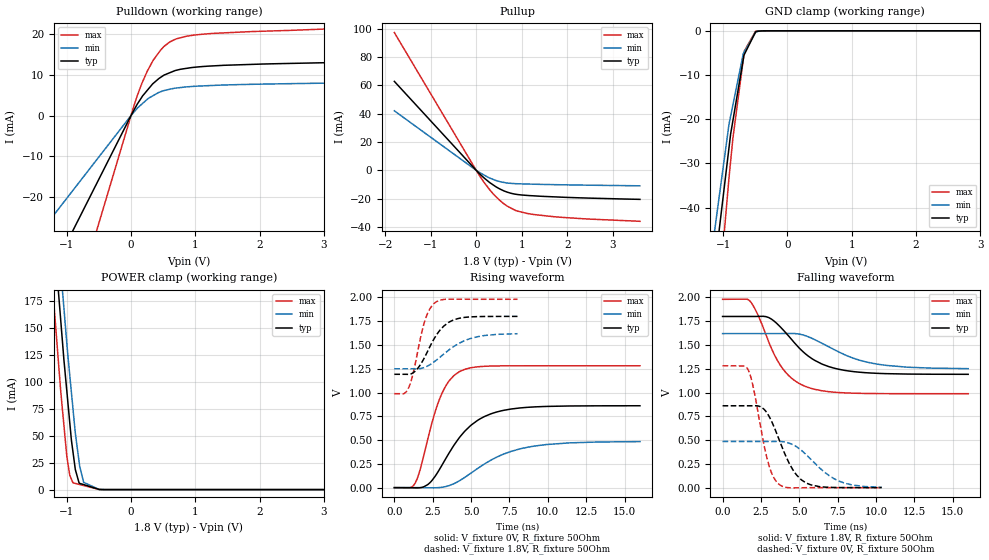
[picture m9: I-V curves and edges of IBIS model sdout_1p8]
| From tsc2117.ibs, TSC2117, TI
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|   sdout_1p8 Model
[Model]   sdout_1p8
Model_type   3-state
Polarity   Non-Inverting
Vmeas = 0.9
Vref = 0.9
Cref = 10pF
Rref = 50
|   typ   min   max
|   (nom PVT)   (fast PVT)   (slow PVT)
|C_comp from frequency sweep method (F=25MHz)
|C_comp   4.331e-12   4.023e-12   4.384e-12
|ON state : BUFFER OUTPUT TURNED HIGH
|C_comp   4.331e-12   4.023e-12   4.384e-12
|OFF state: BUFFER IN HIGH IMPEDANCE
|C_comp   1.705e-12   1.701e-12   1.707e-12
|C_comp from LC tank measurement(L=1nH)
|Resonant Frequency(Hz)   4.060e+09   4.120e+09   4.000e+09
C_comp   1.538e-12   1.494e-12   1.585e-12
|ON state : BUFFER OUTPUT TURNED HIGH
|Resonant Frequency(Hz)   4.060e+09   4.120e+09   4.000e+09
|C_comp   1.538e-12   1.494e-12   1.585e-12
|OFF state: BUFFER IN HIGH IMPEDANCE
|Resonant Frequency(Hz)   4.240e+09   4.260e+09   4.238e+09
|C_comp   1.410e-12   1.397e-12   1.411e-12
| Where nom  PVT is Nominal Process, 1.8V, 48C
|   Fast PVT is Strong Process,  1.98V, -40C
|   Slow PVT is Weak Process,   1.62V, 108C
[Voltage Range]   1.8   1.62   1.98
|Ambient Temperature   25   85   -40
|Junction Temperature
[Temperature Range]   48   108   -40
[Pullup Reference]   1.8   1.62   1.98
[Pulldown Reference]   0   0   0
[Power Clamp Reference]   1.8   1.62   1.98
[GND Clamp Reference]   0   0   0
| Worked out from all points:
|   slope of the pulldown table from 0 to 0.27 V, typ, clamps not added: 41.3 ohm
|   slope of the pullup table from 0 to 0.27 V, typ, clamps not added: 34 ohm
|   GND clamp passes 1 mA (typ) near -0.52 V on its own axis
|   POWER clamp passes 1 mA (typ) near -0.54 V on its own axis
|   falling waveform, V_fixture 1.8V, R_fixture 50Ohm: 20-80 % time 2.48ns typ, 3.15ns min, 1.86ns max; typ from 1.8 V to 1.19 V
|   rising waveform, V_fixture 0V, R_fixture 50Ohm: 20-80 % time 2.4ns typ, 3.26ns min, 1.41ns max; typ from 0 V to 0.861 V
|   rising waveform, V_fixture 1.8V, R_fixture 50Ohm: 20-80 % time 1.33ns typ, 1.97ns min, 843ps max; typ from 1.19 V to 1.8 V
|   falling waveform, V_fixture 0V, R_fixture 50Ohm: 20-80 % time 1.43ns typ, 2.05ns min, 947ps max; typ from 0.861 V to 0 V
[Pulldown]
|   Voltage   I(typ)   I(min)   I(max)
-1.8V     -56.49mA   -36.75mA   -95.55mA
-72mV     -2.259mA   -1.47mA    -3.822mA
95.04mV   2.758mA    1.751mA    4.798mA
168.3mV   4.552mA    2.822mA    7.911mA
251.5mV   6.192mA    3.988mA    10.89mA
348.5mV   7.968mA    4.952mA    13.71mA
463.3mV   9.448mA    5.897mA    16.21mA
601.9mV   10.55mA    6.481mA    18.13mA
698.9mV   11.15mA    6.779mA    18.88mA
855.4mV   11.62mA    7.059mA    19.53mA
1.277V    12.25mA    7.427mA    20.26mA
3.6V      13.28mA    8.129mA    21.69mA
[GND Clamp]
|   Voltage   I(typ)   I(min)   I(max)
-1.8V     -205.1mA   -122.8mA   -348.8mA
-1.168V   -58.11mA   -49.06mA   -76.74mA
-910.4mV  -26.61mA   -21.27mA   -33.47mA
-883.8mV  -23.38mA   -19.33mA   -29.52mA
-847.4mV  -20.24mA   -16.71mA   -24.19mA
-686.9mV  -6.4mA     -5.151mA   -6.472mA
-676.8mV  -5.531mA   -4.896mA   -5.359mA
-669.2mV  -5.311mA   -4.704mA   -4.525mA
-495mV    -237uA     -292.7uA   -66.28uA
-309.4mV  -2.036uA   -3.46uA    -90.99nA
3.6V      0A         0A         0A
[Pullup]
|   Voltage   I(typ)   I(min)   I(max)
-1.8V     62.74mA    41.98mA    97.18mA
95.04mV   -3.093mA   -1.942mA   -4.857mA
348.5mV   -9.775mA   -6.119mA   -15.69mA
601.9mV   -14.42mA   -8.513mA   -23.45mA
683.1mV   -15.42mA   -8.991mA   -25.3mA
900.9mV   -17.04mA   -9.476mA   -28.73mA
1.277V    -18.04mA   -9.812mA   -31.23mA
2.376V    -19.52mA   -10.46mA   -34.22mA
3.6V      -20.5mA    -10.94mA   -35.98mA
[POWER Clamp]
|   Voltage   I(typ)   I(min)   I(max)
-1.8V     718.4mA    754.7mA    668.7mA
-1.215V   248.1mA    295.1mA    184.9mA
-1.131V   185.5mA    231.6mA    120.5mA
-1.044V   121.1mA    169.1mA    60.29mA
-999.9mV  92.81mA    137.3mA    32.12mA
-952.4mV  62.33mA    106.3mA    13.33mA
-902.9mV  35.25mA    75.48mA    6.332mA
-865.8mV  18.64mA    52.58mA    5.764mA
-806.4mV  5.948mA    25.44mA    4.853mA
-737.1mV  4.66mA     6.776mA    3.79mA
-494.1mV  159.6uA    107.3uA    77.17uA
3.6V      0A         0A         0A
[Ramp]
R_load = 50
|   typ   min   max
dV/dt_r   0.516429/2.38634e-09   0.29034/3.24376e-09   0.768595/1.41029e-09
dV/dt_f   0.365028/2.46088e-09   0.22133/3.14467e-09   0.59544/1.85975e-09
[Falling Waveform]
V_fixture = 1.8V
V_fixture_min = 1.62V
V_fixture_max = 1.98V
R_fixture = 50Ohm
|   Time   V(typ)   V(min)   V(max)
0s        1.8V       1.62V      1.98V
1.777ns   1.8V       1.62V      1.963V
2.196ns   1.8V       1.62V      1.853V
3.007ns   1.788V     1.62V      1.533V
3.774ns   1.688V     1.62V      1.284V
4.531ns   1.552V     1.621V     1.146V
5.455ns   1.4V       1.594V     1.061V
7.226ns   1.258V     1.455V     1.004V
9.631ns   1.206V     1.312V     989.8mV
16ns      1.192V     1.251V     987.6mV
[Rising Waveform]
V_fixture = 0V
V_fixture_min = 0V
V_fixture_max = 0V
R_fixture = 50Ohm
|   Time   V(typ)   V(min)   V(max)
0s        2.139nV    8.544nV    632.1pV
1.363ns   -2.152mV   64.27uV    48.91mV
2.186ns   32.98mV    -1.575mV   515.8mV
2.981ns   202.5mV    1.456mV    945.1mV
3.575ns   366.4mV    21.64mV    1.124V
4.301ns   538.9mV    77.96mV    1.224V
5.812ns   742.7mV    242.7mV    1.275V
7.589ns   825.8mV    380mV      1.281V
9.889ns   853.6mV    452.6mV    1.281V
16ns      860.7mV    483.9mV    1.281V
[Rising Waveform]
V_fixture = 1.8V
V_fixture_min = 1.62V
V_fixture_max = 1.98V
R_fixture = 50Ohm
|   Time   V(typ)   V(min)   V(max)
0s        1.191V     1.249V     987.6mV
644ps     1.191V     1.249V     989.3mV
920ps     1.191V     1.249V     1.045V
1.21ns    1.206V     1.249V     1.19V
1.974ns   1.371V     1.264V     1.746V
2.613ns   1.571V     1.325V     1.94V
3.229ns   1.699V     1.405V     1.979V
4.18ns    1.779V     1.514V     1.981V
5.824ns   1.799V     1.598V     1.98V
8.023ns   1.8V       1.618V     1.98V
[Falling Waveform]
V_fixture = 0V
V_fixture_min = 0V
V_fixture_max = 0V
R_fixture = 50Ohm
|   Time   V(typ)   V(min)   V(max)
0s        860.8mV    485.3mV    1.281V
1.683ns   860.8mV    485.3mV    1.234V
1.981ns   860.9mV    485.3mV    1.069V
2.907ns   782.8mV    485.3mV    302.5mV
3.222ns   687.4mV    485.3mV    142.6mV
3.607ns   536.4mV    485.4mV    43.91mV
4.57ns    190.4mV    452.6mV    -2.326mV
5.483ns   46.26mV    341.2mV    -542.3uV
7.677ns   746.2uV    62.62mV    5.544uV
10.37ns   12.11uV    3.499mV    38.83nV
